PROGRAM MAIN
VAR
	el2521_axis:	axis_ref;
	el2521_power:	mc_power;
	el2521_home:	mc_home;
	home_do: BOOL;			(*用HMI中的开关代替*)
	sensor AT %I*: BOOL;	(*EL1004的1通道*)
END_VAR

//使能
el2521_power(Axis:=el2521_axis , Enable:= TRUE, Enable_Positive:=TRUE , Enable_Negative:=TRUE ,  );
//找原点
el2521_home(Axis:=el2521_axis , Execute:= home_do, Position:=0 ,bCalibrationCam:=sensor ,  );

END_PROGRAM
